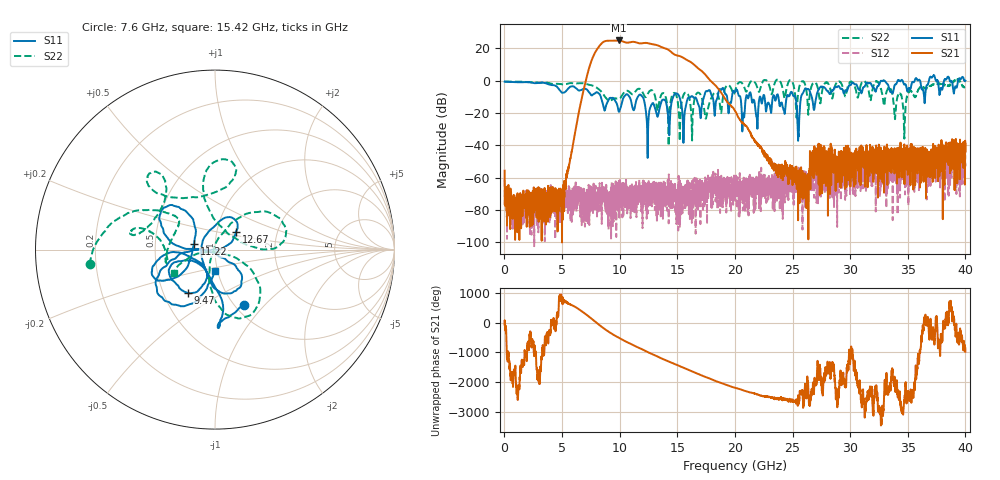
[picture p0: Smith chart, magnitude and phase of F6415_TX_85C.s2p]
!Keysight Technologies,N5245B,MY52451815,A.15.70.20
!Date: Thursday, April 18, 2024 11:16:21
!Correction: S33(C  2-Port  )
!S43(C  2-Port  )
!S34(C  2-Port  )
!S44(C  2-Port  )
!S2P File: Measurements: S33, S43, S34, S44:
# Hz S  RI  R 50
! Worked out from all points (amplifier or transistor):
!   4000 points, 10 MHz to 40 GHz, reference 50 ohm
!   highest |S21| = 24.7 dB at 9.9 GHz (marker M1)
!   |S21| within 3 dB of that: 8.277 GHz to 13.28 GHz (5.003 GHz wide, 46.4 % of centre)
!   unconditionally stable (mu >= 1): start of sweep to 22.47 GHz; 24.89 GHz to 32.86 GHz; 32.97 GHz to 34.13 GHz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
!   at 6.67 GHz: K = 2820.04, MAG = -5.7 dB, |S12| = -75.8 dB
!   at 20.01 GHz: K = 4394.58, MAG = -17.0 dB, |S12| = -64.0 dB
!   at 40 GHz: K = 169.16, MAG = -19.2 dB, |S12| = -51.4 dB
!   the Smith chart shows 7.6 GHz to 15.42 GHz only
!   S11 on the Smith chart (normalised r, x): 7.6 GHz: 1.09, -0.77; 9.47 GHz: 0.66, -0.35; 11.22 GHz: 0.79, +0.05; 12.67 GHz: 1.24, +0.25; 15.42 GHz: 0.97, -0.24
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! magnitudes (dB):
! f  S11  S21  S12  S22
! 10 MHz  -0.8  -55.7  -61.2  -0.6
! 1.06 GHz  -1.0  -76.3  -78.5  -0.7
! 4.88 GHz  -6.7  -76.6  -83.7  -2.2
! 6.68 GHz  -5.9  -11.8  -75.5  -1.6
! 7.6 GHz  -9.2  13.2  -67.6  -3.1
! 9.47 GHz  -10.9  24.6  -87.0  -11.4
! 9.9 GHz  -18.7  24.7  -66.2  -11.4
! 11.22 GHz  -18.4  23.9  -71.4  -8.2
! 12.67 GHz  -16.3  22.7  -69.1  -6.0
! 13.34 GHz  -21.3  21.6  -71.2  -17.4
! 14.92 GHz  -8.0  15.6  -88.6  -9.4
! 15.42 GHz  -18.4  14.4  -71.6  -11.6
! 20.01 GHz  -7.1  -19.0  -64.0  -6.5
! 20.71 GHz  -21.8  -26.5  -63.3  -2.5
! 23.56 GHz  -11.6  -55.2  -67.8  0.0
! 25.03 GHz  -9.0  -55.4  -57.9  -1.7
! 25.51 GHz  -33.2  -55.8  -66.0  -6.7
! 26.24 GHz  -5.3  -58.5  -69.6  -8.0
! 26.67 GHz  -10.2  -46.0  -68.4  -3.2
! 33.34 GHz  -3.7  -45.6  -64.6  -4.5
! 34.69 GHz  -2.5  -44.2  -55.7  -33.9
! 40 GHz  -0.1  -39.1  -51.4  -2.8
